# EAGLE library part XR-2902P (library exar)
MICROCONTROLLER
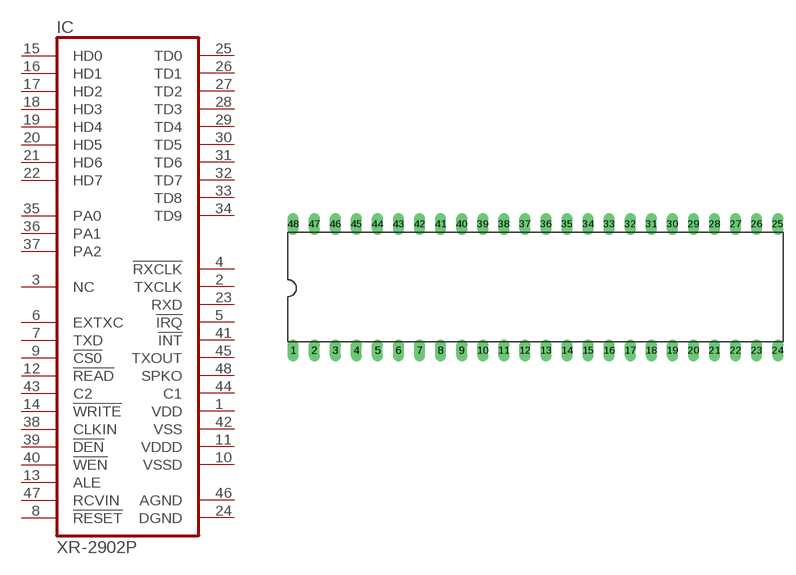
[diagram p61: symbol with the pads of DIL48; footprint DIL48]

Designator prefix IC

## XR-2902P (OC_FARNELL: unknown; OC_NEWARK: unknown)  [DIL48]
1  VDD  pwr
2  TXCLK  out
3  NC  nc
4  !RXCLK  out
5  !IRQ  out
6  EXTXC  in
7  TXD  in
8  !RESET  in
9  !CS0  in
10  VSSD  pwr
11  VDDD  pwr
12  !READ  in
13  ALE  in
14  !WRITE  in
15  HD0
16  HD1
17  HD2
18  HD3
19  HD4
20  HD5
21  HD6
22  HD7
23  RXD  out
24  DGND  pwr
25  TD0
26  TD1
27  TD2
28  TD3
29  TD4
30  TD5
31  TD6
32  TD7
33  TD8
34  TD9
35  PA0
36  PA1
37  PA2
38  CLKIN  in
39  !DEN  in
40  !WEN  in
41  !INT  out
42  VSS  pwr
43  C2  in
44  C1  out
45  TXOUT  out
46  AGND  pwr
47  RCVIN  in
48  SPKO  out

## Footprint DIL48 (pad centres in mm)
Dual In Line Package
drill 0.813 long: 1 -29.21,-7.62; 2 -26.67,-7.62; 3 -24.13,-7.62; 4 -21.59,-7.62; 5 -19.05,-7.62; 6 -16.51,-7.62; 7 -13.97,-7.62; 8 -11.43,-7.62; 9 -8.89,-7.62; 10 -6.35,-7.62; 11 -3.81,-7.62; 12 -1.27,-7.62; 13 1.27,-7.62; 14 3.81,-7.62; 15 6.35,-7.62; 16 8.89,-7.62; 17 11.43,-7.62; 18 13.97,-7.62; 19 16.51,-7.62; 20 19.05,-7.62; 21 21.59,-7.62; 22 24.13,-7.62; 23 26.67,-7.62; 24 29.21,-7.62; 25 29.21,7.62; 26 26.67,7.62; 27 24.13,7.62; 28 21.59,7.62; 29 19.05,7.62; 30 16.51,7.62; 31 13.97,7.62; 32 11.43,7.62; 33 8.89,7.62; 34 6.35,7.62; 35 3.81,7.62; 36 1.27,7.62; 37 -1.27,7.62; 38 -3.81,7.62; 39 -6.35,7.62; 40 -8.89,7.62; 41 -11.43,7.62; 42 -13.97,7.62; 43 -16.51,7.62; 44 -19.05,7.62; 45 -21.59,7.62; 46 -24.13,7.62; 47 -26.67,7.62; 48 -29.21,7.62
